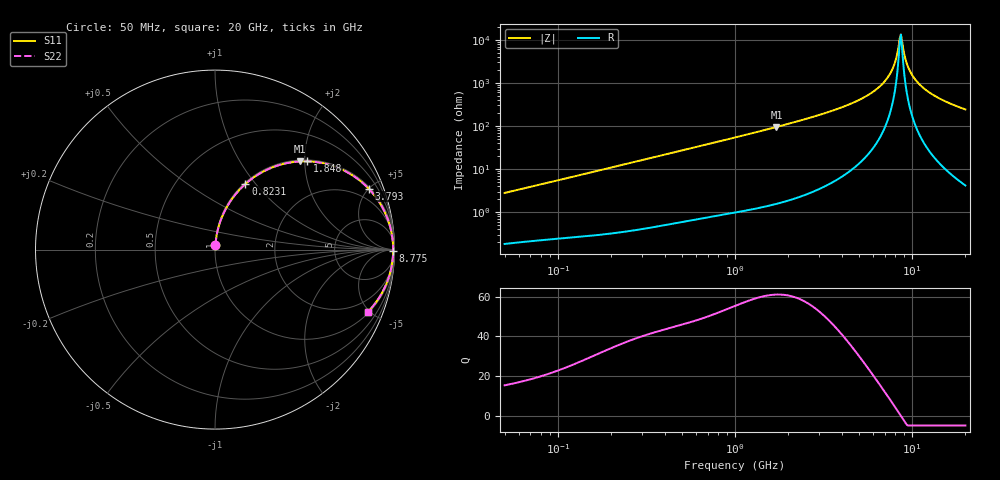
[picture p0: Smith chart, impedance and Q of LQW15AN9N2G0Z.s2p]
!Murata Part Number: LQW15AN9N2G0Z
!These Parameters are Measured in Series Mode Connection
!  o--[Z]--o
!Port1  Port2
!  o-------o
!Freq. Start=50[MHz] Stop=20[GHz], 401[Steps]
# Hz S RI R 50
!Freq.(Hz) S11(Real) S11(Imag) S21(Real) S21(Imag) S12(Real) S12(Imag) S22(Real) S22(Imag)
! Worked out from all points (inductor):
!   401 points, 50 MHz to 20 GHz, reference 50 ohm
!   read as one part in series: L = 8.8 nH near 51.52 MHz
!   highest Q = 61 at 1.715 GHz (marker M1), where L = 8.82 nH
!   self-resonance near 8.516 GHz
!   S11 on the Smith chart (normalised r, x): 50 MHz: 1.00, +0.06; 823.1 MHz: 1.02, +0.89; 1.848 GHz: 1.03, +2.06; 3.793 GHz: 1.12, +4.99; 8.775 GHz: open; 20 GHz: 1.08, -4.85
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5e7  0.0026 0.0277  0.9974 -0.0277  0.9974 -0.0277  0.0026 0.0277
1.364002e8  0.00816 0.0736  0.9918 -0.0736  0.9918 -0.0736  0.00816 0.0736
3.721004e8  0.0431 0.1916  0.9569 -0.1916  0.9569 -0.1916  0.0431 0.1916
8.230629e8  0.1696 0.3658  0.8304 -0.3658  0.8304 -0.3658  0.1696 0.3658
1e9  0.2306 0.4123  0.7694 -0.4123  0.7694 -0.4123  0.2306 0.4123
1.714689e9  0.4748 0.4912  0.5252 -0.4912  0.5252 -0.4912  0.4748 0.4912
1.848039e9  0.5147 0.4916  0.4853 -0.4916  0.4853 -0.4916  0.5147 0.4916
2.728004e9  0.7182 0.4409  0.2818 -0.4409  0.2818 -0.4409  0.7182 0.4409
3.792786e9  0.8561 0.3396  0.1439 -0.3396  0.1439 -0.3396  0.8561 0.3396
4.81993e9  0.926 0.2467  0.074 -0.2467  0.074 -0.2467  0.926 0.2467
5.856089e9  0.9636 0.1657  0.0364 -0.1657  0.0364 -0.1657  0.9636 0.1657
6.701223e9  0.9804 0.1084  0.0196 -0.1084  0.0196 -0.1084  0.9804 0.1084
7.442007e9  0.9884 0.0634  0.0116 -0.0634  0.0116 -0.0634  0.9884 0.0634
8.020766e9  0.9916 0.0312  0.00843 -0.0312  0.00843 -0.0312  0.9916 0.0312
8.516016e9  0.9926 0.00546  0.00742 -0.00546  0.00742 -0.00546  0.9926 0.00546
8.774992e9  0.9926 -0.00743  0.00742 0.00743  0.00742 0.00743  0.9926 -0.00743
9.178299e9  0.992 -0.0268  0.00805 0.0268  0.00805 0.0268  0.992 -0.0268
9.600142e9  0.9906 -0.0461  0.00944 0.0461  0.00944 0.0461  0.9906 -0.0461
1.019291e10  0.9875 -0.0719  0.0125 0.0719  0.0125 0.0719  0.9875 -0.0719
1.098561e10  0.9818 -0.104  0.0182 0.104  0.0182 0.104  0.9818 -0.104
1.396067e10  0.9482 -0.2058  0.0518 0.2058  0.0518 0.2058  0.9482 -0.2058
2e10  0.8505 -0.3481  0.1495 0.3481  0.1495 0.3481  0.8505 -0.3481
